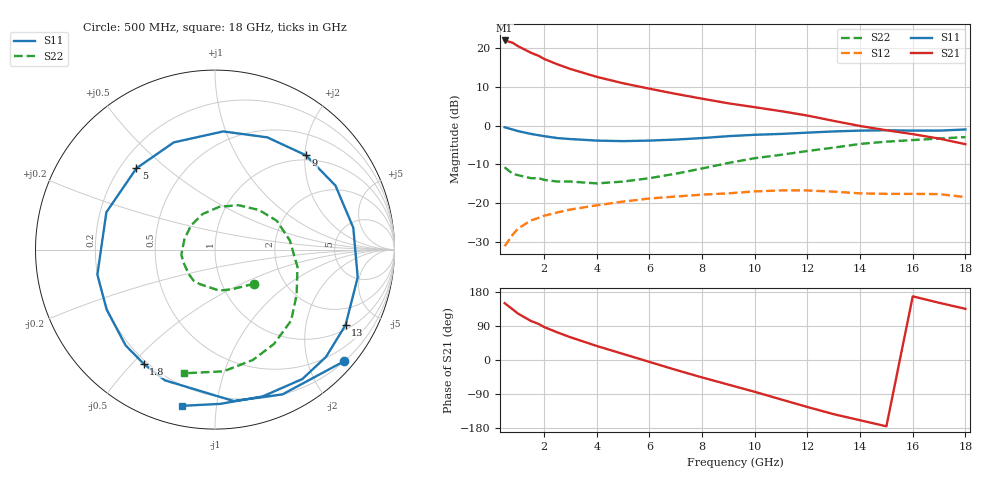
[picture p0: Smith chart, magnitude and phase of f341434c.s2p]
!ATF-34143
!S-PARAMETERS at Vds=4V  Id=60mA.  LAST UPDATED 01-29-99
# ghz s ma r 50
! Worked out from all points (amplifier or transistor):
!   23 points, 500 MHz to 18 GHz, reference 50 ohm
!   highest |S21| = 21.9 dB at 500 MHz (marker M1)
!   |S21| within 3 dB of that: start of sweep to 1.451 GHz
!   unconditionally stable (mu >= 1): 5.195 GHz to end of sweep
!   at 1.5 GHz: K = 0.46, MSG = 21.6 dB, |S12| = -24.4 dB
!   at 7 GHz: K = 1.10, MAG = 11.3 dB, |S12| = -18.3 dB
!   at 18 GHz: K = 1.33, MAG = 3.4 dB, |S12| = -18.4 dB
!   lowest NFmin = 0.11 dB at 500 MHz
!   S11 on the Smith chart (normalised r, x): 500 MHz: 0.21, -2.66; 1.8 GHz: 0.19, -0.54; 5 GHz: 0.27, +0.40; 9 GHz: 0.90, +2.02; 13 GHz: 1.17, -3.35; 18 GHz: 0.10, -0.81
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0.5  0.95 -41.0  12.45 150.0  0.028 68.0  0.29 -41.0
0.8  0.89 -65.0  11.65 134.0  0.039 57.0  0.24 -67.0
1  0.85 -83.0  10.55 123.0  0.047 49.0  0.23 -84.0
1.5  0.78 -111.0  8.646 103.0  0.06 38.0  0.21 -114.0
1.8  0.75 -122.0  7.873 95.0  0.065 33.0  0.21 -125.0
2  0.73 -133.0  7.207 87.0  0.069 29.0  0.2 -136.0
2.5  0.69 -151.0  6.149 73.0  0.076 22.0  0.19 -155.0
3  0.67 -168.0  5.345 60.0  0.083 15.0  0.19 -171.0
4  0.64 161.0  4.232 37.0  0.094 3.0  0.18 162.0
5  0.63 134.0  3.501 16.0  0.105 -10.0  0.19 135.0
6  0.64 111.0  2.983 -5.0  0.115 -24.0  0.21 109.0
7  0.66 86.0  2.557 -26.0  0.122 -38.0  0.24 84.0
8  0.69 65.0  2.217 -46.0  0.129 -51.0  0.28 62.0
9  0.73 46.0  1.932 -65.0  0.134 -65.0  0.33 42.0
10  0.76 28.0  1.723 -84.0  0.142 -79.0  0.38 25.0
11  0.78 9.0  1.531 -104.0  0.146 -94.0  0.42 7.0
12  0.81 -11.0  1.344 -124.0  0.146 -111.0  0.47 -12.0
13  0.84 -30.0  1.148 -143.0  0.141 -126.0  0.52 -29.0
15  0.87 -56.0  0.87 -175.0  0.132 -150.0  0.62 -58.0
16  0.86 -72.0  0.775 168.0  0.132 -163.0  0.65 -71.0
17  0.86 -88.0  0.68 151.0  0.131 -178.0  0.68 -86.0
18  0.89 -102.0  0.575 135.0  0.12 169.0  0.71 -104.0
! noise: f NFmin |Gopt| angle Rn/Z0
0.5  0.11  0.84  15  0.14
0.9  0.14  0.78  30  0.12
1.5  0.2  0.69  53  0.1
1.8  0.23  0.66  62  0.1
2.5  0.33  0.55  91  0.07
3  0.39  0.5  111  0.05
5  0.67  0.39  -173  0.04
6  0.81  0.39  -137  0.07
8  1.1  0.47  -76  0.26
10  1.39  0.62  -37  0.6
